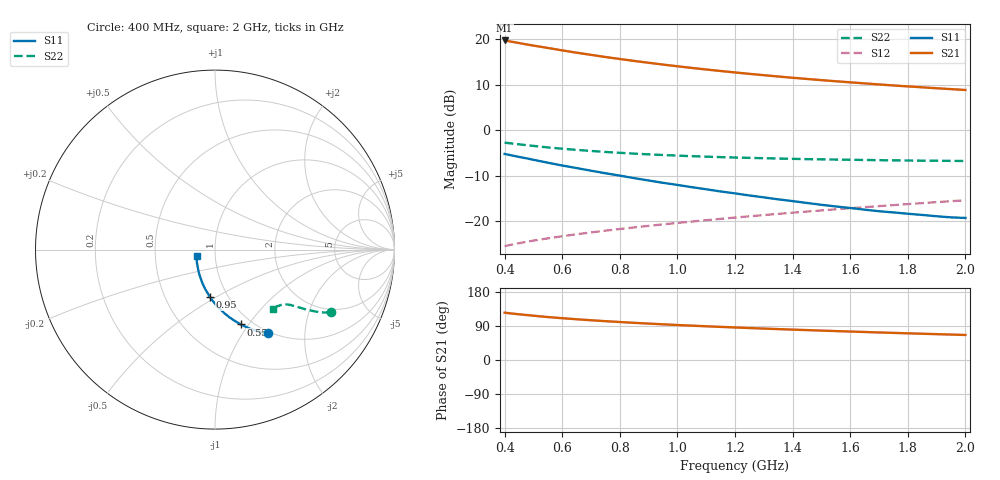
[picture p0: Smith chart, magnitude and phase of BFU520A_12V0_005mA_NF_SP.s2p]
! Filename:  P:\Prog\Test\Noise\ATS_data\Testdata_Net\06 Compressed Noise after Statistics\BFU520A_APG2013_30_A05_12p0V_005mA_NF_CM01_D.sf
! Date/Time: Wed 24/Apr/2013 20:06:21
! BFU520A_APG2013_30_A05_12p0V_1to20mA_NF_CM01_Bias4_R.sf
! Noise Parameter Data File
! BFU520A_APG2013_30_A05_12p0V_1to20mA_NF_CM01
! Date/time: Thu Apr 11 10:46:45 2013
! VAR V_out= 12.001000
! VAR I_out= 5.000000
! VAR V_in= 0.815300
! VAR I_in= 0.048705
! Device data file deembeded for feedlines and parallel
! Original file: \06 Compressed Noise after Statistics\BFU520A_APG2013_30_A05_12p0V_005mA_NF_CM01_R.sf
! Feed-files: PR017V01_150413_Feed1.s2p, PR017V01_150413_Feed2.s2p
! Parallel-file: PR017V01_150413_Par.s2p
# MHz S MA R 50
!  Freq-MHz  S11-mag  S11-arg  S21-mag  S21-arg  S12-mag  S12-arg  S22-mag  S22-arg
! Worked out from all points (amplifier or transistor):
!   37 points, 400 MHz to 2 GHz, reference 50 ohm
!   highest |S21| = 19.8 dB at 400 MHz (marker M1)
!   |S21| within 3 dB of that: start of sweep to 682.9 MHz
!   unconditionally stable (mu >= 1): 1.676 GHz to end of sweep
!   at 500 MHz: K = 0.62, MSG = 21.4 dB, |S12| = -24.2 dB
!   at 1.1 GHz: K = 0.92, MSG = 16.6 dB, |S12| = -19.7 dB
!   at 2 GHz: K = 1.01, MAG = 11.5 dB, |S12| = -15.3 dB
!   lowest NFmin = 0.66 dB at 420 MHz
!   S11 on the Smith chart (normalised r, x): 400 MHz: 0.97, -1.30; 550 MHz: 0.89, -0.92; 950 MHz: 0.83, -0.47; 2 GHz: 0.81, -0.06
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400  0.5514 -57.7  9.72 124.8  0.05351 65.1  0.7336 -28.5
420  0.5353 -59.8  9.468 123.0  0.05523 64.7  0.721 -29.1
440  0.5191 -61.7  9.23 121.4  0.05691 64.4  0.7091 -29.6
480  0.4906 -65.2  8.752 118.4  0.06004 63.8  0.6858 -30.6
500  0.4756 -66.9  8.538 116.9  0.0616 63.6  0.6757 -31.0
550  0.4414 -70.9  8.044 113.3  0.06518 63.2  0.65 -31.9
600  0.4117 -74.6  7.563 110.3  0.06877 63.0  0.6293 -32.6
650  0.3857 -77.9  7.134 107.5  0.07231 62.9  0.6109 -33.2
700  0.361 -81.2  6.753 104.9  0.07576 62.9  0.5944 -33.7
750  0.3384 -84.3  6.397 102.5  0.07917 63.0  0.5798 -34.1
800  0.3185 -87.4  6.082 100.2  0.08261 63.1  0.5671 -34.5
850  0.2989 -90.4  5.792 98.0  0.08602 63.2  0.5555 -34.9
900  0.2818 -93.2  5.527 96.0  0.08946 63.4  0.5455 -35.3
950  0.2656 -95.9  5.283 94.1  0.09285 63.6  0.5363 -35.6
1050  0.238 -101.3  4.853 90.6  0.09973 64.0  0.5209 -36.3
1150  0.2135 -107.0  4.49 87.4  0.1068 64.3  0.5088 -37.0
1200  0.2033 -109.6  4.329 85.9  0.1103 64.5  0.5035 -37.4
1350  0.1749 -118.0  3.906 81.5  0.1211 64.8  0.4907 -38.6
1500  0.1523 -126.9  3.564 77.6  0.1321 65.1  0.4803 -39.9
1650  0.1347 -136.0  3.282 73.9  0.1436 65.2  0.4733 -41.4
1750  0.1256 -143.1  3.116 71.5  0.1511 65.2  0.4684 -42.4
2000  0.1092 -160.5  2.779 66.1  0.1709 65.0  0.4611 -45.4
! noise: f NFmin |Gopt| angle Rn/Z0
400  0.7016  0.2243  13.84  0.1406
460  0.6786  0.2166  17.9  0.1344
600  0.7873  0.2289  20.69  0.1539
800  0.7656  0.177  40.07  0.1198
1000  0.7767  0.1718  49.59  0.1157
1200  0.8109  0.1724  62.03  0.1137
1400  0.8269  0.1473  75.83  0.1056
1600  0.8537  0.1436  89.7  0.0951
1800  0.8315  0.1437  114.9  0.0842
2000  0.8642  0.1465  125.5  0.0816
